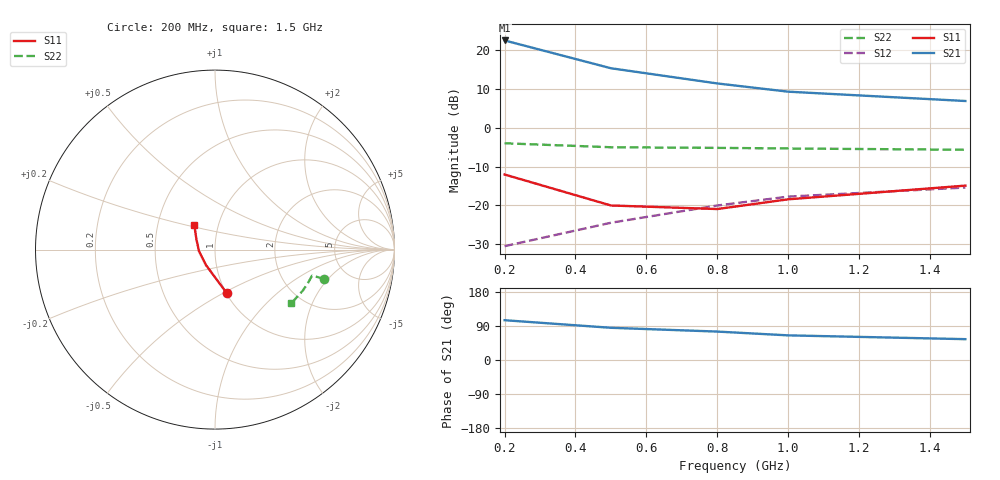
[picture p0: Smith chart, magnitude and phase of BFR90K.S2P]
!  BFR90K.S2P
!  BFR90
!  VCE=10V; IC=30mA
#  GHZ S MA R 50
!  S-PARAMETER DATA
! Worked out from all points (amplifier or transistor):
!   5 points, 200 MHz to 1.5 GHz, reference 50 ohm
!   highest |S21| = 22.4 dB at 200 MHz (marker M1)
!   |S21| within 3 dB of that: start of sweep to 326 MHz
!   unconditionally stable (mu >= 1): 327.1 MHz to end of sweep
!   at 200 MHz: K = 0.91, MSG = 26.4 dB, |S12| = -30.5 dB
!   at 800 MHz: K = 1.07, MAG = 14.0 dB, |S12| = -20.0 dB
!   at 1.5 GHz: K = 1.05, MAG = 9.8 dB, |S12| = -15.4 dB
0.2  0.25 -75.0  13.2 105.0  0.03 75.0  0.63 -15.0
0.5  0.1 -120.0  5.8 85.0  0.06 75.0  0.56 -15.0
0.8  0.09 -175.0  3.7 75.0  0.1 75.0  0.55 -20.0
1  0.12 150.0  2.9 65.0  0.13 75.0  0.54 -25.0
1.5  0.18 130.0  2.2 55.0  0.17 70.0  0.52 -35.0
